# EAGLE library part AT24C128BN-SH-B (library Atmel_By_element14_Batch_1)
Two-wire Serial EEPROM
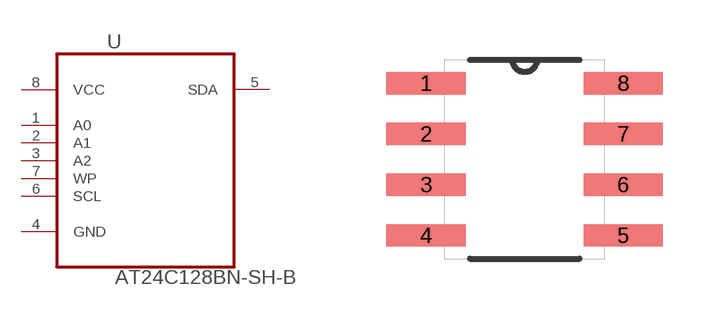
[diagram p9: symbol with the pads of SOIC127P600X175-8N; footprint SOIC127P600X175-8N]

Designator prefix U

## AT24C128BN-SH-B (MPN: AT24C128BN-SH-B; OC_FARNELL: 1362649; OC_NEWARK: 50M3322; PACKAGE: SOIC-8; SUPPLIER: Atmel)  [SOIC127P600X175-8N]
1  A0  in
2  A1  in
3  A2  in
4  GND  pas
5  SDA
6  SCL  in
7  WP  in
8  VCC  pwr

## Footprint SOIC127P600X175-8N (pad centres in mm)
smd 1.981 x 0.559: 1 -2.464,1.905; 2 -2.464,0.635; 3 -2.464,-0.635; 4 -2.464,-1.905; 5 2.464,-1.905; 6 2.464,-0.635; 7 2.464,0.635; 8 2.464,1.905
